| IBIS file generated by  Version 3.24
|   DRA78x_abf
[IBIS ver]   5.0
[File name]   DRA78x_abf.ibs
[File Rev]   1.1.2
[Date]   Tue Aug 30, 2016, 13:57:0
[Source]   Data created at Texas Instruments
[Notes]   DRA78x 15mm IBIS Model Revision History
   Version 1.1.2, August 30th, 2016
   - Combined DDR selectors for similiar signals
   - Modified model names for easier selection
   Version 1.1.1, January 15th, 2015
   - Assign DDR_CK and DDR_NCK as differential pair
   Version 1.1.0, November 7th, 2014
   - Added support for DDR2 and LPDDR2
   Version 1.0.0, May 22, 2014
   - Initial Release
   Note 1) Checked by IBISCHK5.
   Note 2) Interfaces Included in this IBIS Model
   - VIP
   - DPI
   - CAM
   - CPI
   - CSI2
   - EMIF
   - GPMC
   - TIMER
   - I2C
   - UART
   - MCSPI
   - QSPI
   - MCASP
   - DCAN
   - GMAC
   - EMMC
   - GPIO
   - PWM
   - DEBUG
[Disclaimer] Please be aware that in the absence of a written agreement,
   Texas Instruments (TI) assumes no liability for: 1) the
   accuracy of the IBIS models provided to your company, 2) the
   proper functioning of these IBIS models in your design or for
   any resulting applications, or, 3) infringement of patents,
   copyrights, or intellectual property rights resulting from
   your use of these IBIS models. TI provides IBIS models as a
   service to our customers and therefore reserves the right to
   limit distribution of the IBIS models.
[Copyright]   Property of Texas Instruments Incorporated. Unauthorised
   reproduction and/or distribution is strictly prohibited. This
   product is protected under copyright law and trade secret law
   as an unpublished work. Created 2013,(C) Copyright 2013,
   Texas Instruments Incorporated., All Rights Reserved. These
   commodities are under the U.S. Government distribution license
   control.As such,they are not to be re-exported without the
   prior approval of the U.S. Department of Commerce.
|   Component DRA78x_abf
[Component]   DRA78x_abf
[Manufacturer]   Texas Instruments.
| Source IO level model revisions
|Model   Revision   Date
|DDR_DIFFIOPB_V   2.5   23 May 2014
|BC1833DV40DCPBFBP1811_SSCEV   2.0   Sep 11, 2013
|IHHV1833DVHYP1811_SSCEV   1.0   Dec 24, 2012
|BI2C1833DVFZP18_SSCEV   2.0   Sep 11, 2013
|BC1833DV40DCPBFBP1811_SSCEH   2.0   Sep 11, 2013
|CAMERARX_CORE   0.9   March 31, 2014
|DDR_SEIOPB_V   2.5   23 May 2014
|IQ1833DVTCKPBFBP18LL_SSCEV   2.0   Sep 11, 2013
|CAMERARX_ADDON   0.9   March 31, 2014
[Package]
|   typ   min   max
R_pkg   0.667349380701754   64.242E-3   1671.14E-3
L_pkg   3.85005961842105E-009 0.900514E-9   6.82372E-9
C_pkg   5.31210293859649E-013 0.214455E-12   0.846797E-12
[Pin]   signal_name   model_name   R_pin   L_pin   C_pin
P19   ADC_IN6   NC
M22   ADC_IN3   NC
M19   ADC_IN0   NC
P20   ADC_VREFP   NC
M20   ADC_IN1   NC
N22   ADC_IN4   NC
N21   ADC_IN5   NC
M21   ADC_IN2   NC
P18   ADC_IN7   NC
A21   ATESTV   NC
A16   CSI2_0_DX4   Selector_14  866.498E-3 4.24036E-9 0.371535E-12
A15   CSI2_0_DX3   Selector_14  824.084E-3 4.09623E-9 0.353901E-12
B12   CSI2_0_DY1   Selector_7   880.169E-3 3.81411E-9 0.40211E-12
A13   CSI2_0_DX2   Selector_5   917.025E-3 4.11456E-9 0.365851E-12
B15   CSI2_0_DY3   Selector_8   864.002E-3 3.95726E-9 0.383183E-12
B11   CSI2_0_DY0   Selector_8   881.601E-3 3.85263E-9 0.418142E-12
B13   CSI2_0_DY2   Selector_7   810.956E-3 3.78817E-9 0.380345E-12
A12   CSI2_0_DX1   Selector_5   842.043E-3 3.90631E-9 0.371721E-12
A11   CSI2_0_DX0   Selector_14  843.258E-3 3.98139E-9 0.381546E-12
B16   CSI2_0_DY4   Selector_8   880.712E-3 4.08429E-9 0.380274E-12
P17   CVIDEO_VFB   NC
T17   CVIDEO_TVOUT   NC
T18   CVIDEO_RSET   NC
N5   DCAN1_TX   Selector_9   221.153E-3 2.4896E-9  0.508994E-12
N6   DCAN1_RX   Selector_9   174.193E-3 2.2145E-9  0.51767E-12
W6   DCAN2_RX   Selector_4   404.154E-3 4.83175E-9 0.778223E-12
W7   DCAN2_TX   Selector_4   192.368E-3 2.60394E-9 0.469083E-12
W22   DDR1_D30   Selector_3   1303.09E-3 4.54181E-9 0.726069E-12
Y5   DDR1_D5   Selector_3   1117.89E-3 4.60346E-9 0.559528E-12
F1   DDR1_RASN   Selector_11  1296.71E-3 4.52967E-9 0.754591E-12
Y2   DDR1_D22   Selector_3   1482.08E-3 6.2409E-9  0.654749E-12
AB9   DDR1_ECC_D7   Selector_3   1318.63E-3 4.88449E-9 0.563531E-12
W21   DDR1_DQM3   Selector_11  1456.76E-3 4.87842E-9 0.653267E-12
R2   DDR1_A14   Selector_11  1366.99E-3 5.45703E-9 0.784996E-12
U20   DDR1_D27   Selector_3   1251.59E-3 4.23052E-9 0.739335E-12
Y21   DDR1_D9   Selector_3   1410.24E-3 6.0268E-9  0.671587E-12
AA4   DDR1_D6   Selector_3   1162.31E-3 4.7233E-9  0.543846E-12
D2   DDR1_BA2   Selector_11  1345.76E-3 5.19955E-9 0.639721E-12
Y1   DDR1_D23   Selector_3   1408.11E-3 6.15406E-9 0.588347E-12
R22   DDR1_D28   Selector_3   1320.57E-3 4.76807E-9 0.489006E-12
AA9   DDR1_ECC_D6   Selector_3   1365.05E-3 4.86342E-9 0.607781E-12
AA6   DDR1_D0   Selector_3   1059.66E-3 3.64899E-9 0.498846E-12
T22   DDR1_DQSN3   Selector_13  1213.01E-3 5.45946E-9 0.503501E-12
U4   DDR1_A0   Selector_11  1344.44E-3 4.91464E-9 0.702976E-12
N2   DDR1_A7   Selector_11  1428.38E-3 4.75993E-9 0.706672E-12
C3   DDR1_A13   Selector_11  1361.06E-3 5.06314E-9 0.799988E-12
AA21   DDR1_D10   Selector_3   1467.96E-3 6.31542E-9 0.547716E-12
AA8   DDR1_D1   Selector_3   945.134E-3 3.4619E-9  0.630603E-12
AA7   DDR1_D3   Selector_3   957.149E-3 3.58448E-9 0.583994E-12
AB11   DDR1_ECC_D5   Selector_3   1288.72E-3 4.87133E-9 0.699912E-12
AB3   DDR1_DQM2   Selector_11  1231.76E-3 5.08662E-9 0.503327E-12
Y3   DDR1_D18   Selector_3   1232.03E-3 4.85881E-9 0.631657E-12
F3   DDR1_CKE0   Selector_11  1309.3E-3  4.76705E-9 0.661629E-12
AB5   DDR1_DQSN0   Selector_13  1049.22E-3 4.99231E-9 0.470641E-12
D3   DDR1_A2   Selector_11  1451.79E-3 5.79785E-9 0.671604E-12
Y9   DDR1_ECC_D3   Selector_3   1229.56E-3 4.83423E-9 0.735586E-12
AA19   DDR1_D12   Selector_3   1439.57E-3 5.39046E-9 0.68973E-12
V1   DDR1_A15   Selector_11  1671.14E-3 6.82372E-9 0.584748E-12
Y22   DDR1_D11   Selector_3   1477.72E-3 5.88672E-9 0.66686E-12
AA2   DDR1_D17   Selector_3   1345.48E-3 5.16009E-9 0.660701E-12
C1   DDR1_A1   Selector_11  1461.14E-3 6.3818E-9  0.45563E-12
R4   DDR1_A3   Selector_11  1197.34E-3 4.46899E-9 0.55908E-12
AB4   DDR1_D4   Selector_3   1257.55E-3 5.2014E-9  0.502406E-12
AA3   DDR1_D16   Selector_3   1260.55E-3 5.10575E-9 0.591139E-12
AA5   DDR1_DQS0   Selector_15  1095.27E-3 5.06071E-9 0.461046E-12
U3   DDR1_D20   Selector_3   1373.61E-3 5.35193E-9 0.615526E-12
AA13   DDR1_ECC_D4   Selector_3   1323.91E-3 4.88968E-9 0.72932E-12
R3   DDR1_A11   Selector_11  1401.24E-3 5.13832E-9 0.846797E-12
AA10   DDR1_DQS_ECC   Selector_15  1216.87E-3 5.36065E-9 0.556044E-12
D1   DDR1_A10   Selector_11  1329.72E-3 5.13668E-9 0.654383E-12
Y20   DDR1_DQSN1   Selector_13  1342.47E-3 5.82752E-9 0.510552E-12
U22   DDR1_D31   Selector_3   1275.16E-3 4.04716E-9 0.698905E-12
B3   DDR1_BA0   Selector_11  1400.57E-3 6.05502E-9 0.525495E-12
Y11   DDR1_ECC_D0   Selector_3   1389.08E-3 4.76944E-9 0.677831E-12
G2   DDR1_NCK   Selector_12  1342.99E-3 5.99964E-9 0.561576E-12
G1   DDR1_CK   Selector_10  1310.97E-3 5.71231E-9 0.561547E-12
AB20   DDR1_D13   Selector_3   1411.85E-3 5.50356E-9 0.654257E-12
E3   DDR1_WEN   Selector_11  1243.69E-3 4.61238E-9 0.658685E-12
T1   DDR1_A8   Selector_11  1304.21E-3 4.85445E-9 0.734575E-12
V2   DDR1_D19   Selector_3   1371.08E-3 5.42143E-9 0.606473E-12
U2   DDR1_A12   Selector_11  1542.41E-3 5.63849E-9 0.829165E-12
AA12   DDR1_ECC_D1   Selector_3   1144.49E-3 4.56631E-9 0.700588E-12
Y8   DDR1_D2   Selector_3   1013.88E-3 3.94703E-9 0.557904E-12
AA20   DDR1_DQS1   Selector_15  1228.33E-3 5.79816E-9 0.471177E-12
AA11   DDR1_ECC_D2   Selector_3   1220.61E-3 4.58017E-9 0.693337E-12
T21   DDR1_DQS3   Selector_15  1153.95E-3 5.24704E-9 0.550448E-12
Y6   DDR1_D7   Selector_3   1093.76E-3 4.50306E-9 0.494525E-12
V20   DDR1_D29   Selector_3   1164.32E-3 4.20118E-9 0.57292E-12
A3   DDR1_BA1   Selector_11  1458.59E-3 5.71787E-9 0.715307E-12
R21   DDR1_D26   Selector_3   1257.83E-3 5.0006E-9  0.530122E-12
AB18   DDR1_D15   Selector_3   1249.3E-3  4.97423E-9 0.581239E-12
T2   DDR1_A6   Selector_11  1416.66E-3 5.20489E-9 0.708511E-12
Y18   DDR1_DQM1   Selector_11  1284.23E-3 4.79732E-9 0.50954E-12
V3   DDR1_D21   Selector_3   1264.57E-3 4.95585E-9 0.550028E-12
Y17   DDR1_D14   Selector_3   1330.64E-3 5.30397E-9 0.518058E-12
AB10   DDR1_DQSN_ECC   Selector_13  1157.81E-3 5.29728E-9 0.552246E-12
W1   DDR1_DQS2   Selector_15  1243.23E-3 6.03074E-9 0.523353E-12
F2   DDR1_CASN   Selector_11  1359.06E-3 4.84573E-9 0.69557E-12
N3   DDR1_A5   Selector_11  1256.87E-3 4.88274E-9 0.822611E-12
T4   DDR1_A4   Selector_11  1225.96E-3 4.48501E-9 0.686864E-12
N1   DDR1_RST   Selector_11  1200.46E-3 4.86402E-9 0.785997E-12
T20   DDR1_D25   Selector_3   1192.14E-3 4.07414E-9 0.613975E-12
P2   DDR1_ODT0   Selector_11  1319.42E-3 4.7618E-9  0.67937E-12
B2   DDR1_CSN0   Selector_11  1118.13E-3 4.60514E-9 0.624304E-12
U1   DDR1_A9   Selector_11  1430.76E-3 5.46625E-9 0.726337E-12
AB8   DDR1_DQM0   Selector_11  1220.87E-3 4.17469E-9 0.549437E-12
W2   DDR1_DQSN2   Selector_13  1247.14E-3 6.0081E-9  0.5286E-12
U21   DDR1_D24   Selector_3   1331.68E-3 4.36055E-9 0.733678E-12
AB13   DDR1_DQM_ECC   Selector_11  1291.15E-3 4.6118E-9  0.626638E-12
AA18   DDR1_D8   Selector_3   1418.02E-3 5.43567E-9 0.642913E-12
H1   EMU0   Selector_9   346.558E-3 3.945E-9   0.481326E-12
H2   EMU1   Selector_9   273.662E-3 3.26523E-9 0.455933E-12
C8   GPMC_CS6   Selector_4   284.574E-3 3.07589E-9 0.456596E-12
B4   GPMC_AD14   Selector_4   370.025E-3 4.53157E-9 0.506776E-12
F8   GPMC_AD2   Selector_4   247.733E-3 2.79628E-9 0.40664E-12
A5   GPMC_AD9   Selector_4   420.627E-3 4.64798E-9 0.533623E-12
D10   GPMC_CS2   Selector_4   187.985E-3 2.10165E-9 0.402136E-12
A4   GPMC_AD15   Selector_4   397.46E-3  4.86112E-9 0.54337E-12
A10   GPMC_OEN_REN   Selector_4   373.838E-3 3.74242E-9 0.451922E-12
C12   GPMC_CLK   Selector_4   326.387E-3 3.50172E-9 0.618617E-12
E8   GPMC_AD0   Selector_4   267.003E-3 2.80033E-9 0.441078E-12
D8   GPMC_WAIT0   Selector_4   266.22E-3  2.88134E-9 0.40446E-12
D6   GPMC_AD10   Selector_4   221.234E-3 2.54407E-9 0.422159E-12
C10   GPMC_CS0   Selector_4   311.079E-3 3.00524E-9 0.44399E-12
E12   GPMC_BEN1   Selector_4   320.958E-3 3.02188E-9 0.594246E-12
A6   GPMC_AD4   Selector_4   437.778E-3 4.50088E-9 0.532669E-12
D12   GPMC_BEN0   Selector_4   292.929E-3 3.06566E-9 0.606716E-12
D7   GPMC_AD13   Selector_4   304.94E-3  3.19335E-9 0.404685E-12
C6   GPMC_AD7   Selector_4   318.071E-3 3.30116E-9 0.469481E-12
F7   GPMC_AD5   Selector_4   185.525E-3 2.0225E-9  0.416218E-12
C5   GPMC_AD11   Selector_4   325.471E-3 3.54687E-9 0.491936E-12
F10   GPMC_CS5   Selector_4   64.242E-3  0.900514E-9 0.269895E-12
F12   GPMC_ADVN_ALE   Selector_4   266.228E-3 3.02405E-9 0.433779E-12
B9   GPMC_CS4   Selector_4   335.103E-3 3.42038E-9 0.495123E-12
B10   GPMC_WEN   Selector_4   347.42E-3  3.76872E-9 0.466852E-12
B6   GPMC_AD8   Selector_4   330.979E-3 3.67024E-9 0.516724E-12
A7   GPMC_AD1   Selector_4   356.051E-3 4.20904E-9 0.431934E-12
B5   GPMC_AD12   Selector_4   348.127E-3 3.95513E-9 0.545603E-12
E7   GPMC_AD6   Selector_4   170.88E-3  1.99455E-9 0.378953E-12
B7   GPMC_AD3   Selector_4   324.465E-3 3.66337E-9 0.443124E-12
A9   GPMC_CS3   Selector_4   361.691E-3 3.93006E-9 0.505481E-12
E10   GPMC_CS1   Selector_4   175.122E-3 1.66792E-9 0.3576E-12
L3   I2C1_SCL   Selector_6   253.012E-3 2.73735E-9 0.427091E-12
L6   I2C2_SCL   Selector_6   75.9648E-3 0.951563E-9 0.319419E-12
L5   I2C2_SDA   Selector_6   125.18E-3  1.32917E-9 0.429362E-12
L4   I2C1_SDA   Selector_6   200.127E-3 2.27796E-9 0.471893E-12
B17   MDIO_D   Selector_4   344.949E-3 4.04087E-9 0.518979E-12
B19   MDIO_MCLK   Selector_4   350.85E-3  4.29974E-9 0.567622E-12
G5   NMIN   Selector_2   206.034E-3 2.38103E-9 0.441195E-12
G3   PORZ   Selector_16  262.543E-3 3.23109E-9 0.436378E-12
G4   RESETN   Selector_2   221.901E-3 2.67053E-9 0.416783E-12
F17   RGMII0_TXD0   Selector_4   190.61E-3  2.90538E-9 0.453282E-12
E17   RGMII0_TXD1   Selector_4   243.515E-3 2.63118E-9 0.416182E-12
C16   RGMII0_TXC   Selector_4   241.728E-3 2.9564E-9  0.393586E-12
A20   RGMII0_RXD0   Selector_4   378.744E-3 5.06456E-9 0.540103E-12
D16   RGMII0_TXD2   Selector_4   272.921E-3 3.27597E-9 0.364109E-12
C18   RGMII0_RXCTL   Selector_4   334.922E-3 3.70159E-9 0.476584E-12
B18   RGMII0_RXC   Selector_4   383.991E-3 4.38625E-9 0.584646E-12
C17   RGMII0_TXCTL   Selector_4   299.95E-3  3.2778E-9  0.45012E-12
A19   RGMII0_RXD3   Selector_4   382.21E-3  4.86108E-9 0.516381E-12
C20   RGMII0_RXD1   Selector_4   337.059E-3 4.59601E-9 0.437991E-12
B20   RGMII0_RXD2   Selector_4   337.895E-3 4.50338E-9 0.543729E-12
E16   RGMII0_TXD3   Selector_4   258.565E-3 2.83197E-9 0.371553E-12
F4   RSTOUTN   Selector_17  380.521E-3 4.67151E-9 0.614741E-12
J6   RTCK   Selector_17  116.119E-3 1.272E-9   0.297361E-12
T5   SPI1_D0   Selector_9   400.982E-3 4.51214E-9 0.798667E-12
M2   SPI1_SCLK   Selector_9   267.537E-3 2.74861E-9 0.533728E-12
U6   SPI1_D1   Selector_9   264.657E-3 3.64443E-9 0.560725E-12
R5   SPI1_CS1   Selector_9   343.795E-3 3.60294E-9 0.730371E-12
R6   SPI1_CS0   Selector_9   184.528E-3 2.64387E-9 0.507092E-12
L2   SPI2_CS0   Selector_9   258.507E-3 3.05366E-9 0.398683E-12
N4   SPI2_D1   Selector_9   159.815E-3 1.82356E-9 0.50115E-12
L1   SPI2_SCLK   Selector_9   350.336E-3 3.8191E-9  0.466382E-12
R7   SPI2_D0   Selector_9   194.814E-3 2.55749E-9 0.476249E-12
J2   TCLK   Selector_1   254.697E-3 3.15214E-9 0.378464E-12
J1   TDI   Selector_2   326.413E-3 3.56361E-9 0.460549E-12
J4   TDO   Selector_17  149.34E-3  1.81311E-9 0.321612E-12
J3   TMS   Selector_2   263.583E-3 2.96504E-9 0.445849E-12
J5   TRSTN   Selector_2   140.82E-3  1.56546E-9 0.304121E-12
C14   UART1_RTSN   Selector_4   271.077E-3 3.37526E-9 0.592546E-12
E14   UART1_TXD   Selector_4   264.17E-3  3.29024E-9 0.580159E-12
F14   UART1_CTSN   Selector_4   186.167E-3 2.17244E-9 0.522293E-12
F13   UART1_RXD   Selector_4   183.573E-3 2.09803E-9 0.458722E-12
F16   UART2_RTSN   Selector_4   324.1E-3   3.89433E-9 0.569445E-12
D14   UART2_RXD   Selector_4   355.638E-3 3.93152E-9 0.716287E-12
F15   UART2_CTSN   Selector_4   294.057E-3 3.59825E-9 0.5892E-12
D15   UART2_TXD   Selector_4   282.377E-3 3.48879E-9 0.582841E-12
G18   VIN1A_D0   Selector_9   243.254E-3 2.85171E-9 0.501809E-12
K21   VIN1A_D10   Selector_9   305.782E-3 3.65235E-9 0.458586E-12
G19   VIN1A_VSYNC0   Selector_9   246.63E-3  3.12189E-9 0.492055E-12
J17   VIN1A_D8   Selector_9   228.648E-3 2.7531E-9  0.442602E-12
K17   VIN1A_D12   Selector_9   176.785E-3 2.20565E-9 0.388461E-12
G21   VIN1A_D1   Selector_9   363.135E-3 4.19976E-9 0.575956E-12
F22   VIN1A_CLK0   Selector_9   392.642E-3 4.6109E-9  0.584552E-12
K22   VIN1A_D9   Selector_9   322.551E-3 4.1764E-9  0.421938E-12
H22   VIN1A_D6   Selector_9   377.875E-3 4.39918E-9 0.51729E-12
G22   VIN1A_D2   Selector_9   377.7E-3   4.53068E-9 0.560377E-12
K18   VIN1A_D11   Selector_9   140.113E-3 1.67467E-9 0.346405E-12
F19   VIN1A_HSYNC0   Selector_9   284.459E-3 3.30938E-9 0.524099E-12
K19   VIN1A_D13   Selector_9   199.308E-3 2.30236E-9 0.395571E-12
K20   VIN1A_D14   Selector_9   225.717E-3 2.61957E-9 0.370053E-12
H19   VIN1A_D5   Selector_9   237.915E-3 2.77378E-9 0.458354E-12
F20   VIN1A_FLD0   Selector_9   301.259E-3 3.71239E-9 0.51085E-12
L21   VIN1A_D15   Selector_9   299.827E-3 3.51197E-9 0.45532E-12
F21   VIN1A_DE0   Selector_9   358.032E-3 4.33398E-9 0.519573E-12
H20   VIN1A_D4   Selector_9   261.044E-3 3.17335E-9 0.468927E-12
H21   VIN1A_D7   Selector_9   336.581E-3 3.95216E-9 0.508497E-12
H18   VIN1A_D3   Selector_9   318.602E-3 3.64388E-9 0.577444E-12
M18   VIN2A_FLD0   Selector_9   107.879E-3 1.39908E-9 0.25939E-12
M17   VIN2A_DE0   Selector_9   69.4518E-3 0.993642E-9 0.214455E-12
L22   VIN2A_CLK0   Selector_9   326.657E-3 4.13124E-9 0.457766E-12
U15   VOUT1_D2   Selector_4   188.192E-3 2.06593E-9 0.524972E-12
U17   VOUT1_DE   Selector_4   180.267E-3 2.5353E-9  0.421769E-12
W8   VOUT1_D21   Selector_4   286.194E-3 3.22952E-9 0.660641E-12
W9   VOUT1_D19   Selector_4   176.719E-3 2.32055E-9 0.469196E-12
W11   VOUT1_D17   Selector_4   170.859E-3 1.88713E-9 0.475399E-12
U13   VOUT1_D10   Selector_4   121.41E-3  1.22509E-9 0.414317E-12
V9   VOUT1_D18   Selector_4   188.281E-3 2.08068E-9 0.521271E-12
AB17   VOUT1_CLK   Selector_4   365.568E-3 4.16017E-9 0.565211E-12
U9   VOUT1_D16   Selector_4   183.337E-3 2.11554E-9 0.534405E-12
AA15   VOUT1_D6   Selector_4   388.553E-3 3.79821E-9 0.620296E-12
AA17   VOUT1_HSYNC   Selector_4   406.915E-3 4.58133E-9 0.582066E-12
W16   VOUT1_D0   Selector_4   249.496E-3 2.74357E-9 0.544844E-12
AB15   VOUT1_D7   Selector_4   407.232E-3 4.46019E-9 0.539498E-12
AA14   VOUT1_D8   Selector_4   343.58E-3  3.34818E-9 0.554761E-12
W13   VOUT1_D13   Selector_4   238.288E-3 2.20297E-9 0.483663E-12
W15   VOUT1_D5   Selector_4   270.299E-3 2.89534E-9 0.543448E-12
W17   VOUT1_FLD   Selector_4   392.595E-3 4.29688E-9 0.619062E-12
AB14   VOUT1_D9   Selector_4   375.782E-3 3.99293E-9 0.57511E-12
U11   VOUT1_D14   Selector_4   91.4322E-3 0.938044E-9 0.395492E-12
Y15   VOUT1_D4   Selector_4   275.703E-3 3.09509E-9 0.440349E-12
V16   VOUT1_D1   Selector_4   249.155E-3 2.69511E-9 0.49623E-12
Y13   VOUT1_D12   Selector_4   243.754E-3 2.47516E-9 0.457168E-12
V11   VOUT1_D15   Selector_4   146.232E-3 1.44691E-9 0.461628E-12
U16   VOUT1_VSYNC   Selector_4   221.18E-3  2.43907E-9 0.495724E-12
V7   VOUT1_D23   Selector_4   193.825E-3 2.65994E-9 0.580721E-12
U7   VOUT1_D22   Selector_4   185.923E-3 2.5291E-9  0.426436E-12
V13   VOUT1_D11   Selector_4   106.384E-3 1.20262E-9 0.365368E-12
V15   VOUT1_D3   Selector_4   172.909E-3 2.04259E-9 0.422534E-12
U8   VOUT1_D20   Selector_4   165.759E-3 2.12333E-9 0.545066E-12
B21   XI_OSC1   NC
E22   XI_OSC0   NC
C21   XO_OSC1   NC
D22   XO_OSC0   NC
M1   XREF_CLK0   Selector_9   330.711E-3 3.47713E-9 0.50945E-12
[Diff Pin] inv_pin vdiff tdelay_typ tdelay_min tdelay_max
|Differential signal data for cell CAMERARX_ADDON
|CSI2_0_DX3   CSI2_0_DY3
A15   B15   200m   NA
|CSI2_0_DX4   CSI2_0_DY4
A16   B16   200m   NA
|CSI2_0_DX0   CSI2_0_DY0
A11   B11   200m   NA
|Differential signal data for cell CAMERARX_CORE
|CSI2_0_DX1   CSI2_0_DY1
A12   B12   200m   NA
|CSI2_0_DX2   CSI2_0_DY2
A13   B13   200m   NA
|Differential signal data for cell DDR_DIFFIOPB_V
|DDR1_DQS1   DDR1_DQSN1
AA20   Y20   200m   0
|DDR1_DQS_ECC   DDR1_DQSN_ECC
AA10   AB10   200m   0
|DDR1_CK   DDR1_NCK
G1   G2   200m   0
|DDR1_DQS3   DDR1_DQSN3
T21   T22   200m   0
|DDR1_DQS0   DDR1_DQSN0
AA5   AB5   200m   0
|DDR1_DQS2   DDR1_DQSN2
W1   W2   200m   0
|   Usage INPUT#1.8/3.3###IQ1833DVTCKPBFBP18LL_SSCEV.PAD
|   Base model IQ1833DVTCKPBFBP18LL_SSCEV
[Model Selector] Selector_1
IQ1833_V_10P_1P8_M#1 INPUT,1.8V,1.8V MODE,IND,10 PERCENT%,IQ1833_V_10P_1P8
IQ1833_V_5P_1P8_M#2 INPUT,1.8V,1.8V MODE,IND,5 PERCENT%,IQ1833_V_5P_1P8
IQ1833_V_10P_3P3_M#3 INPUT,3.3V,3.3V MODE,IND,10 PERCENT%,IQ1833_V_10P_3P3
IQ1833_V_5P_3P3_M#4 INPUT,3.3V,3.3V MODE,IND,5 PERCENT%,IQ1833_V_5P_3P3
|   Usage INPUT#1.8/3.3###BC1833DV40DCPBFBP1811_SSCEV.PAD
|   Base model BC1833DV40DCPBFBP1811_SSCEV
[Model Selector] Selector_2
BC40D_V_10P_!SC1_1P8_M#194 I/O,1.8V,40D CLASS MODE FAST MODE,IND,10 PERCENT%,BC40D_V_10P_!SC1_1P8
BC40D_V_10P_SC1_1P8_M#195 I/O,1.8V,40C CLASS MODE SLOW MODE,IND,10 PERCENT%,BC40D_V_10P_SC1_1P8
BC40D_V_5P_!SC1_1P8_M#196 I/O,1.8V,40D CLASS MODE FAST MODE,IND,5 PERCENT%,BC40D_V_5P_!SC1_1P8
BC40D_V_5P_SC1_1P8_M#197 I/O,1.8V,40C CLASS MODE SLOW MODE,IND,5 PERCENT%,BC40D_V_5P_SC1_1P8
BC40D_V_10P_!SC1_3P3_M#198 I/O,3.3V,40D CLASS MODE FAST MODE,IND,10 PERCENT%,BC40D_V_10P_!SC1_3P3
BC40D_V_10P_SC1_3P3_M#199 I/O,3.3V,40C CLASS MODE SLOW MODE,IND,10 PERCENT%,BC40D_V_10P_SC1_3P3
BC40D_V_5P_!SC1_3P3_M#200 I/O,3.3V,40D CLASS MODE FAST MODE,IND,5 PERCENT%,BC40D_V_5P_!SC1_3P3
BC40D_V_5P_SC1_3P3_M#201 I/O,3.3V,40C CLASS MODE SLOW MODE,IND,5 PERCENT%,BC40D_V_5P_SC1_3P3
|   Usage I/O#1.2/1.35/1.5/1.8###DDR_SEIOPB_V.PAD
|   Base model DDR_SEIOPB_V
[Model Selector] Selector_3
SR000_DRV48_1P8_M#100 I/O,1.8V,SR000_DRV48_1P8
SR011_DRV40_1P8_M#101 I/O,1.8V,SR011_DRV40_1P8
SR010_DRV40_1P8_M#102 I/O,1.8V,SR010_DRV40_1P8
SR101_DRV40_1P8_M#103 I/O,1.8V,SR101_DRV40_1P8
SR100_DRV40_1P8_M#104 I/O,1.8V,SR100_DRV40_1P8
SR110_DRV40_1P8_M#105 I/O,1.8V,SR110_DRV40_1P8
SR111_DRV40_1P8_M#106 I/O,1.8V,SR111_DRV40_1P8
SR001_DRV40_1P8_M#107 I/O,1.8V,SR001_DRV40_1P8
SR000_DRV40_1P8_M#108 I/O,1.8V,SR000_DRV40_1P8
SR011_DRV34_1P8_M#109 I/O,1.8V,SR011_DRV34_1P8
SR010_DRV34_1P8_M#110 I/O,1.8V,SR010_DRV34_1P8
SR101_DRV34_1P8_M#111 I/O,1.8V,SR101_DRV34_1P8
SR100_DRV34_1P8_M#112 I/O,1.8V,SR100_DRV34_1P8
SR110_DRV34_1P8_M#113 I/O,1.8V,SR110_DRV34_1P8
SR111_DRV34_1P8_M#114 I/O,1.8V,SR111_DRV34_1P8
SR001_DRV34_1P8_M#115 I/O,1.8V,SR001_DRV34_1P8
SR000_DRV34_1P8_M#116 I/O,1.8V,SR000_DRV34_1P8
DDR3_ODT_80_1P5_M#117 INPUT,1.5V,DDR3_ODT_80_1P5
DDR3_ODT_60_1P5_M#118 INPUT,1.5V,DDR3_ODT_60_1P5
DDR3_ODT_120_1P5_M#119 INPUT,1.5V,DDR3_ODT_120_1P5
DDR3L_ODT_80_1P35_M#120 INPUT,1.35V,DDR3L_ODT_80_1P35
DDR3L_ODT_60_1P35_M#121 INPUT,1.35V,DDR3L_ODT_60_1P35
DDR3L_ODT_120_1P35_M#122 INPUT,1.35V,DDR3L_ODT_120_1P35
DDR2_ODT_120_1P8_M#123 INPUT,1.8V,DDR2_ODT_120_1P8
DDR2_ODT_80_1P8_M#124 INPUT,1.8V,DDR2_ODT_80_1P8
DDR2_ODT_60_1P8_M#125 INPUT,1.8V,DDR2_ODT_60_1P8
SR011_DRV40_1P5_M#126 I/O,1.5V,SR011_DRV40_1P5
SR010_DRV40_1P5_M#127 I/O,1.5V,SR010_DRV40_1P5
SR101_DRV40_1P5_M#128 I/O,1.5V,SR101_DRV40_1P5
SR100_DRV40_1P5_M#129 I/O,1.5V,SR100_DRV40_1P5
SR011_DRV60_1P2_M#13 I/O,1.2V,SR011_DRV60_1P2
SR110_DRV40_1P5_M#130 I/O,1.5V,SR110_DRV40_1P5
SR111_DRV40_1P5_M#131 I/O,1.5V,SR111_DRV40_1P5
SR001_DRV40_1P5_M#132 I/O,1.5V,SR001_DRV40_1P5
SR000_DRV40_1P5_M#133 I/O,1.5V,SR000_DRV40_1P5
SR011_DRV34_1P5_M#134 I/O,1.5V,SR011_DRV34_1P5
SR010_DRV34_1P5_M#135 I/O,1.5V,SR010_DRV34_1P5
SR101_DRV34_1P5_M#136 I/O,1.5V,SR101_DRV34_1P5
SR100_DRV34_1P5_M#137 I/O,1.5V,SR100_DRV34_1P5
SR110_DRV34_1P5_M#138 I/O,1.5V,SR110_DRV34_1P5
SR111_DRV34_1P5_M#139 I/O,1.5V,SR111_DRV34_1P5
SR010_DRV60_1P2_M#14 I/O,1.2V,SR010_DRV60_1P2
SR001_DRV34_1P5_M#140 I/O,1.5V,SR001_DRV34_1P5
SR000_DRV34_1P5_M#141 I/O,1.5V,SR000_DRV34_1P5
SR011_DRV48_1P5_M#142 I/O,1.5V,SR011_DRV48_1P5
SR010_DRV48_1P5_M#143 I/O,1.5V,SR010_DRV48_1P5
SR101_DRV48_1P5_M#144 I/O,1.5V,SR101_DRV48_1P5
SR100_DRV48_1P5_M#145 I/O,1.5V,SR100_DRV48_1P5
SR110_DRV48_1P5_M#146 I/O,1.5V,SR110_DRV48_1P5
SR111_DRV48_1P5_M#147 I/O,1.5V,SR111_DRV48_1P5
SR001_DRV48_1P5_M#148 I/O,1.5V,SR001_DRV48_1P5
SR000_DRV48_1P5_M#149 I/O,1.5V,SR000_DRV48_1P5
SR101_DRV60_1P2_M#15 I/O,1.2V,SR101_DRV60_1P2
SR011_DRV40_1P35_M#150 I/O,1.35V,SR011_DRV40_1P35
SR010_DRV40_1P35_M#151 I/O,1.35V,SR010_DRV40_1P35
SR101_DRV40_1P35_M#152 I/O,1.35V,SR101_DRV40_1P35
SR100_DRV40_1P35_M#153 I/O,1.35V,SR100_DRV40_1P35
SR110_DRV40_1P35_M#154 I/O,1.35V,SR110_DRV40_1P35
SR111_DRV40_1P35_M#155 I/O,1.35V,SR111_DRV40_1P35
SR001_DRV40_1P35_M#156 I/O,1.35V,SR001_DRV40_1P35
SR000_DRV40_1P35_M#157 I/O,1.35V,SR000_DRV40_1P35
SR011_DRV34_1P35_M#158 I/O,1.35V,SR011_DRV34_1P35
SR010_DRV34_1P35_M#159 I/O,1.35V,SR010_DRV34_1P35
SR100_DRV60_1P2_M#16 I/O,1.2V,SR100_DRV60_1P2
SR101_DRV34_1P35_M#160 I/O,1.35V,SR101_DRV34_1P35
SR100_DRV34_1P35_M#161 I/O,1.35V,SR100_DRV34_1P35
SR110_DRV34_1P35_M#162 I/O,1.35V,SR110_DRV34_1P35
SR111_DRV34_1P35_M#163 I/O,1.35V,SR111_DRV34_1P35
SR001_DRV34_1P35_M#164 I/O,1.35V,SR001_DRV34_1P35
SR000_DRV34_1P35_M#165 I/O,1.35V,SR000_DRV34_1P35
SR011_DRV48_1P35_M#166 I/O,1.35V,SR011_DRV48_1P35
SR010_DRV48_1P35_M#167 I/O,1.35V,SR010_DRV48_1P35
SR101_DRV48_1P35_M#168 I/O,1.35V,SR101_DRV48_1P35
SR100_DRV48_1P35_M#169 I/O,1.35V,SR100_DRV48_1P35
SR110_DRV60_1P2_M#17 I/O,1.2V,SR110_DRV60_1P2
SR110_DRV48_1P35_M#170 I/O,1.35V,SR110_DRV48_1P35
SR111_DRV48_1P35_M#171 I/O,1.35V,SR111_DRV48_1P35
SR001_DRV48_1P35_M#172 I/O,1.35V,SR001_DRV48_1P35
SR000_DRV48_1P35_M#173 I/O,1.35V,SR000_DRV48_1P35
SR111_DRV60_1P2_M#18 I/O,1.2V,SR111_DRV60_1P2
SR001_DRV60_1P2_M#19 I/O,1.2V,SR001_DRV60_1P2
SR000_DRV60_1P2_M#20 I/O,1.2V,SR000_DRV60_1P2
SR011_DRV80_1P2_M#29 I/O,1.2V,SR011_DRV80_1P2
SR010_DRV80_1P2_M#30 I/O,1.2V,SR010_DRV80_1P2
SR101_DRV80_1P2_M#31 I/O,1.2V,SR101_DRV80_1P2
SR100_DRV80_1P2_M#32 I/O,1.2V,SR100_DRV80_1P2
SR110_DRV80_1P2_M#33 I/O,1.2V,SR110_DRV80_1P2
SR111_DRV80_1P2_M#34 I/O,1.2V,SR111_DRV80_1P2
SR001_DRV80_1P2_M#35 I/O,1.2V,SR001_DRV80_1P2
SR000_DRV80_1P2_M#36 I/O,1.2V,SR000_DRV80_1P2
SR011_DRV40_1P2_M#45 I/O,1.2V,SR011_DRV40_1P2
SR010_DRV40_1P2_M#46 I/O,1.2V,SR010_DRV40_1P2
SR101_DRV40_1P2_M#47 I/O,1.2V,SR101_DRV40_1P2
SR100_DRV40_1P2_M#48 I/O,1.2V,SR100_DRV40_1P2
SR110_DRV40_1P2_M#49 I/O,1.2V,SR110_DRV40_1P2
SR111_DRV40_1P2_M#50 I/O,1.2V,SR111_DRV40_1P2
SR001_DRV40_1P2_M#51 I/O,1.2V,SR001_DRV40_1P2
SR000_DRV40_1P2_M#52 I/O,1.2V,SR000_DRV40_1P2
SR011_DRV34_1P2_M#53 I/O,1.2V,SR011_DRV34_1P2
SR010_DRV34_1P2_M#54 I/O,1.2V,SR010_DRV34_1P2
SR101_DRV34_1P2_M#55 I/O,1.2V,SR101_DRV34_1P2
SR100_DRV34_1P2_M#56 I/O,1.2V,SR100_DRV34_1P2
SR110_DRV34_1P2_M#57 I/O,1.2V,SR110_DRV34_1P2
SR111_DRV34_1P2_M#58 I/O,1.2V,SR111_DRV34_1P2
SR001_DRV34_1P2_M#59 I/O,1.2V,SR001_DRV34_1P2
SR000_DRV34_1P2_M#60 I/O,1.2V,SR000_DRV34_1P2
SR011_DRV48_1P2_M#77 I/O,1.2V,SR011_DRV48_1P2
SR010_DRV48_1P2_M#78 I/O,1.2V,SR010_DRV48_1P2
SR101_DRV48_1P2_M#79 I/O,1.2V,SR101_DRV48_1P2
SR100_DRV48_1P2_M#80 I/O,1.2V,SR100_DRV48_1P2
SR110_DRV48_1P2_M#81 I/O,1.2V,SR110_DRV48_1P2
SR111_DRV48_1P2_M#82 I/O,1.2V,SR111_DRV48_1P2
SR001_DRV48_1P2_M#83 I/O,1.2V,SR001_DRV48_1P2
SR000_DRV48_1P2_M#84 I/O,1.2V,SR000_DRV48_1P2
SR011_DRV48_1P8_M#93 I/O,1.8V,SR011_DRV48_1P8
SR010_DRV48_1P8_M#94 I/O,1.8V,SR010_DRV48_1P8
SR101_DRV48_1P8_M#95 I/O,1.8V,SR101_DRV48_1P8
SR100_DRV48_1P8_M#96 I/O,1.8V,SR100_DRV48_1P8
SR110_DRV48_1P8_M#97 I/O,1.8V,SR110_DRV48_1P8
SR111_DRV48_1P8_M#98 I/O,1.8V,SR111_DRV48_1P8
SR001_DRV48_1P8_M#99 I/O,1.8V,SR001_DRV48_1P8
|   Usage I/O#1.8/3.3###BC1833DV40DCPBFBP1811_SSCEH.PAD
|   Base model BC1833DV40DCPBFBP1811_SSCEH
[Model Selector] Selector_4
BC40D_H_10P_!SC1_1P8_M#182 I/O,1.8V,40D CLASS MODE FAST MODE,IND,10 PERCENT%,BC40D_H_10P_!SC1_1P8
BC40D_H_10P_SC1_1P8_M#183 I/O,1.8V,40C CLASS MODE SLOW MODE,IND,10 PERCENT%,BC40D_H_10P_SC1_1P8
BC40D_H_5P_!SC1_1P8_M#184 I/O,1.8V,40D CLASS MODE FAST MODE,IND,5 PERCENT%,BC40D_H_5P_!SC1_1P8
BC40D_H_5P_SC1_1P8_M#185 I/O,1.8V,40C CLASS MODE SLOW MODE,IND,5 PERCENT%,BC40D_H_5P_SC1_1P8
BC40D_H_10P_!SC1_3P3_M#186 I/O,3.3V,40D CLASS MODE FAST MODE,IND,10 PERCENT%,BC40D_H_10P_!SC1_3P3
BC40D_H_10P_SC1_3P3_M#187 I/O,3.3V,40C CLASS MODE SLOW MODE,IND,10 PERCENT%,BC40D_H_10P_SC1_3P3
BC40D_H_5P_!SC1_3P3_M#188 I/O,3.3V,40D CLASS MODE FAST MODE,IND,5 PERCENT%,BC40D_H_5P_!SC1_3P3
BC40D_H_5P_SC1_3P3_M#189 I/O,3.3V,40C CLASS MODE SLOW MODE,IND,5 PERCENT%,BC40D_H_5P_SC1_3P3
|   Usage INPUT#1.8###CAMERARX_CORE.PADP
|   Base model CAMERARX_CORE
[Model Selector] Selector_5
CAMERARX_CORE_HSRX_M#176 INPUT,1.8V,CAMERARX_CORE_HSRX
CAMERARX_CORE_LPRX_M#177 INPUT,1.8V,CAMERARX_CORE_LPRX
CAMERARX_CORE_ULPRX_M#178 INPUT,1.8V,CAMERARX_CORE_ULPRX
CAMERARX_CORE_PD_ON_M#179 INPUT,1.8V,CAMERARX_CORE_PD_ON
CAMERARX_CORE_PU_ON_M#180 INPUT,1.8V,CAMERARX_CORE_PU_ON
CAMERARX_CORE_PUPD0_M#181 INPUT,1.8V,CAMERARX_CORE_PUPD0
|   Usage I/O#1.8/3.3###BI2C1833DVFZP18_SSCEV.PAD
|   Base model BI2C1833DVFZP18_SSCEV
[Model Selector] Selector_6
FAST_STD_MODE_1.8V_10P_1P8_M#190 I/O_OPEN_DRAIN,1.8V,FAST MODE AND STD MODE,IND,10 PERCENT%,FAST_STD_MODE_1.8V_10P_1P8
FAST_STD_MODE_3.3V_10P_3P3_M#191 I/O_OPEN_DRAIN,3.3V,FAST MODE AND STD MODE,IND,10 PERCENT%,FAST_STD_MODE_3.3V_10P_3P3
FAST_STD_MODE_1.8V_5P_1P8_M#192 I/O_OPEN_DRAIN,1.8V,FAST MODE AND STD MODE,IND,5 PERCENT%,FAST_STD_MODE_1.8V_5P_1P8
FAST_STD_MODE_3.3V_5P_3P3_M#193 I/O_OPEN_DRAIN,3.3V,FAST MODE AND STD MODE,IND,5 PERCENT%,FAST_STD_MODE_3.3V_5P_3P3
|   Usage INPUT#1.8###CAMERARX_CORE.PADN
|   Base model CAMERARX_CORE
[Model Selector] Selector_7
CAMERARX_CORE_HSRX_M#176 INPUT,1.8V,CAMERARX_CORE_HSRX
CAMERARX_CORE_LPRX_M#177 INPUT,1.8V,CAMERARX_CORE_LPRX
CAMERARX_CORE_ULPRX_M#178 INPUT,1.8V,CAMERARX_CORE_ULPRX
CAMERARX_CORE_PD_ON_M#179 INPUT,1.8V,CAMERARX_CORE_PD_ON
CAMERARX_CORE_PU_ON_M#180 INPUT,1.8V,CAMERARX_CORE_PU_ON
CAMERARX_CORE_PUPD0_M#181 INPUT,1.8V,CAMERARX_CORE_PUPD0
|   Usage INPUT#1.8###CAMERARX_ADDON.PADN
|   Base model CAMERARX_ADDON
[Model Selector] Selector_8
CAMERARX_ADDON_PD_ON_M#10 INPUT,1.8V,CAMERARX_ADDON_PD_ON
CAMERARX_ADDON_PU_ON_M#11 INPUT,1.8V,CAMERARX_ADDON_PU_ON
CAMERARX_ADDON_PUPD0_M#12 INPUT,1.8V,CAMERARX_ADDON_PUPD0
CAMERARX_ADDON_HSRX_M#7 INPUT,1.8V,CAMERARX_ADDON_HSRX
CAMERARX_ADDON_LPRX_M#8 INPUT,1.8V,CAMERARX_ADDON_LPRX
CAMERARX_ADDON_ULPRX_M#9 INPUT,1.8V,CAMERARX_ADDON_ULPRX
|   Usage I/O#1.8/3.3###BC1833DV40DCPBFBP1811_SSCEV.PAD
|   Base model BC1833DV40DCPBFBP1811_SSCEV
[Model Selector] Selector_9
BC40D_V_10P_!SC1_1P8_M#194 I/O,1.8V,40D CLASS MODE FAST MODE,IND,10 PERCENT%,BC40D_V_10P_!SC1_1P8
BC40D_V_10P_SC1_1P8_M#195 I/O,1.8V,40C CLASS MODE SLOW MODE,IND,10 PERCENT%,BC40D_V_10P_SC1_1P8
BC40D_V_5P_!SC1_1P8_M#196 I/O,1.8V,40D CLASS MODE FAST MODE,IND,5 PERCENT%,BC40D_V_5P_!SC1_1P8
BC40D_V_5P_SC1_1P8_M#197 I/O,1.8V,40C CLASS MODE SLOW MODE,IND,5 PERCENT%,BC40D_V_5P_SC1_1P8
BC40D_V_10P_!SC1_3P3_M#198 I/O,3.3V,40D CLASS MODE FAST MODE,IND,10 PERCENT%,BC40D_V_10P_!SC1_3P3
BC40D_V_10P_SC1_3P3_M#199 I/O,3.3V,40C CLASS MODE SLOW MODE,IND,10 PERCENT%,BC40D_V_10P_SC1_3P3
BC40D_V_5P_!SC1_3P3_M#200 I/O,3.3V,40D CLASS MODE FAST MODE,IND,5 PERCENT%,BC40D_V_5P_!SC1_3P3
BC40D_V_5P_SC1_3P3_M#201 I/O,3.3V,40C CLASS MODE SLOW MODE,IND,5 PERCENT%,BC40D_V_5P_SC1_3P3
|   Usage OUTPUT#1.2/1.35/1.5/1.8###DDR_DIFFIOPB_V.PADP
|   Base model DDR_DIFFIOPB_V
[Model Selector] Selector_10
SR011_DRV60_1P2_M#202 I/O,1.2V,SR011_DRV60_1P2
SR010_DRV60_1P2_M#203 I/O,1.2V,SR010_DRV60_1P2
SR101_DRV60_1P2_M#204 I/O,1.2V,SR101_DRV60_1P2
SR100_DRV60_1P2_M#205 I/O,1.2V,SR100_DRV60_1P2
SR110_DRV60_1P2_M#206 I/O,1.2V,SR110_DRV60_1P2
SR111_DRV60_1P2_M#207 I/O,1.2V,SR111_DRV60_1P2
SR001_DRV60_1P2_M#208 I/O,1.2V,SR001_DRV60_1P2
SR000_DRV60_1P2_M#209 I/O,1.2V,SR000_DRV60_1P2
SR011_DRV80_1P2_M#218 I/O,1.2V,SR011_DRV80_1P2
SR010_DRV80_1P2_M#219 I/O,1.2V,SR010_DRV80_1P2
SR101_DRV80_1P2_M#220 I/O,1.2V,SR101_DRV80_1P2
SR100_DRV80_1P2_M#221 I/O,1.2V,SR100_DRV80_1P2
SR110_DRV80_1P2_M#222 I/O,1.2V,SR110_DRV80_1P2
SR111_DRV80_1P2_M#223 I/O,1.2V,SR111_DRV80_1P2
SR001_DRV80_1P2_M#224 I/O,1.2V,SR001_DRV80_1P2
SR000_DRV80_1P2_M#225 I/O,1.2V,SR000_DRV80_1P2
SR011_DRV40_1P2_M#234 I/O,1.2V,SR011_DRV40_1P2
SR010_DRV40_1P2_M#235 I/O,1.2V,SR010_DRV40_1P2
SR101_DRV40_1P2_M#236 I/O,1.2V,SR101_DRV40_1P2
SR100_DRV40_1P2_M#237 I/O,1.2V,SR100_DRV40_1P2
SR110_DRV40_1P2_M#238 I/O,1.2V,SR110_DRV40_1P2
SR111_DRV40_1P2_M#239 I/O,1.2V,SR111_DRV40_1P2
SR001_DRV40_1P2_M#240 I/O,1.2V,SR001_DRV40_1P2
SR000_DRV40_1P2_M#241 I/O,1.2V,SR000_DRV40_1P2
SR011_DRV34_1P2_M#242 I/O,1.2V,SR011_DRV34_1P2
SR010_DRV34_1P2_M#243 I/O,1.2V,SR010_DRV34_1P2
SR101_DRV34_1P2_M#244 I/O,1.2V,SR101_DRV34_1P2
SR100_DRV34_1P2_M#245 I/O,1.2V,SR100_DRV34_1P2
SR110_DRV34_1P2_M#246 I/O,1.2V,SR110_DRV34_1P2
SR111_DRV34_1P2_M#247 I/O,1.2V,SR111_DRV34_1P2
SR001_DRV34_1P2_M#248 I/O,1.2V,SR001_DRV34_1P2
SR000_DRV34_1P2_M#249 I/O,1.2V,SR000_DRV34_1P2
SR011_DRV48_1P2_M#266 I/O,1.2V,SR011_DRV48_1P2
SR010_DRV48_1P2_M#267 I/O,1.2V,SR010_DRV48_1P2
SR101_DRV48_1P2_M#268 I/O,1.2V,SR101_DRV48_1P2
SR100_DRV48_1P2_M#269 I/O,1.2V,SR100_DRV48_1P2
SR110_DRV48_1P2_M#270 I/O,1.2V,SR110_DRV48_1P2
SR111_DRV48_1P2_M#271 I/O,1.2V,SR111_DRV48_1P2
SR001_DRV48_1P2_M#272 I/O,1.2V,SR001_DRV48_1P2
SR000_DRV48_1P2_M#273 I/O,1.2V,SR000_DRV48_1P2
SR011_DRV48_1P8_M#282 I/O,1.8V,SR011_DRV48_1P8
SR010_DRV48_1P8_M#283 I/O,1.8V,SR010_DRV48_1P8
SR101_DRV48_1P8_M#284 I/O,1.8V,SR101_DRV48_1P8
SR100_DRV48_1P8_M#285 I/O,1.8V,SR100_DRV48_1P8
SR110_DRV48_1P8_M#286 I/O,1.8V,SR110_DRV48_1P8
SR111_DRV48_1P8_M#287 I/O,1.8V,SR111_DRV48_1P8
SR001_DRV48_1P8_M#288 I/O,1.8V,SR001_DRV48_1P8
SR000_DRV48_1P8_M#289 I/O,1.8V,SR000_DRV48_1P8
SR011_DRV40_1P8_M#290 I/O,1.8V,SR011_DRV40_1P8
SR010_DRV40_1P8_M#291 I/O,1.8V,SR010_DRV40_1P8
SR101_DRV40_1P8_M#292 I/O,1.8V,SR101_DRV40_1P8
SR100_DRV40_1P8_M#293 I/O,1.8V,SR100_DRV40_1P8
SR110_DRV40_1P8_M#294 I/O,1.8V,SR110_DRV40_1P8
SR111_DRV40_1P8_M#295 I/O,1.8V,SR111_DRV40_1P8
SR001_DRV40_1P8_M#296 I/O,1.8V,SR001_DRV40_1P8
SR000_DRV40_1P8_M#297 I/O,1.8V,SR000_DRV40_1P8
SR011_DRV34_1P8_M#298 I/O,1.8V,SR011_DRV34_1P8
SR010_DRV34_1P8_M#299 I/O,1.8V,SR010_DRV34_1P8
SR101_DRV34_1P8_M#300 I/O,1.8V,SR101_DRV34_1P8
SR100_DRV34_1P8_M#301 I/O,1.8V,SR100_DRV34_1P8
SR110_DRV34_1P8_M#302 I/O,1.8V,SR110_DRV34_1P8
SR111_DRV34_1P8_M#303 I/O,1.8V,SR111_DRV34_1P8
SR001_DRV34_1P8_M#304 I/O,1.8V,SR001_DRV34_1P8
SR000_DRV34_1P8_M#305 I/O,1.8V,SR000_DRV34_1P8
SR011_DRV40_1P5_M#315 I/O,1.5V,SR011_DRV40_1P5
SR010_DRV40_1P5_M#316 I/O,1.5V,SR010_DRV40_1P5
SR101_DRV40_1P5_M#317 I/O,1.5V,SR101_DRV40_1P5
SR100_DRV40_1P5_M#318 I/O,1.5V,SR100_DRV40_1P5
SR110_DRV40_1P5_M#319 I/O,1.5V,SR110_DRV40_1P5
SR111_DRV40_1P5_M#320 I/O,1.5V,SR111_DRV40_1P5
SR001_DRV40_1P5_M#321 I/O,1.5V,SR001_DRV40_1P5
SR000_DRV40_1P5_M#322 I/O,1.5V,SR000_DRV40_1P5
SR011_DRV34_1P5_M#323 I/O,1.5V,SR011_DRV34_1P5
SR010_DRV34_1P5_M#324 I/O,1.5V,SR010_DRV34_1P5
SR101_DRV34_1P5_M#325 I/O,1.5V,SR101_DRV34_1P5
SR100_DRV34_1P5_M#326 I/O,1.5V,SR100_DRV34_1P5
SR110_DRV34_1P5_M#327 I/O,1.5V,SR110_DRV34_1P5
SR111_DRV34_1P5_M#328 I/O,1.5V,SR111_DRV34_1P5
SR001_DRV34_1P5_M#329 I/O,1.5V,SR001_DRV34_1P5
SR000_DRV34_1P5_M#330 I/O,1.5V,SR000_DRV34_1P5
SR011_DRV48_1P5_M#331 I/O,1.5V,SR011_DRV48_1P5
SR010_DRV48_1P5_M#332 I/O,1.5V,SR010_DRV48_1P5
SR101_DRV48_1P5_M#333 I/O,1.5V,SR101_DRV48_1P5
SR100_DRV48_1P5_M#334 I/O,1.5V,SR100_DRV48_1P5
SR110_DRV48_1P5_M#335 I/O,1.5V,SR110_DRV48_1P5
SR111_DRV48_1P5_M#336 I/O,1.5V,SR111_DRV48_1P5
SR001_DRV48_1P5_M#337 I/O,1.5V,SR001_DRV48_1P5
SR000_DRV48_1P5_M#338 I/O,1.5V,SR000_DRV48_1P5
SR011_DRV40_1P35_M#339 I/O,1.35V,SR011_DRV40_1P35
SR010_DRV40_1P35_M#340 I/O,1.35V,SR010_DRV40_1P35
SR101_DRV40_1P35_M#341 I/O,1.35V,SR101_DRV40_1P35
SR100_DRV40_1P35_M#342 I/O,1.35V,SR100_DRV40_1P35
SR110_DRV40_1P35_M#343 I/O,1.35V,SR110_DRV40_1P35
SR111_DRV40_1P35_M#344 I/O,1.35V,SR111_DRV40_1P35
SR001_DRV40_1P35_M#345 I/O,1.35V,SR001_DRV40_1P35
SR000_DRV40_1P35_M#346 I/O,1.35V,SR000_DRV40_1P35
SR011_DRV34_1P35_M#347 I/O,1.35V,SR011_DRV34_1P35
SR010_DRV34_1P35_M#348 I/O,1.35V,SR010_DRV34_1P35
SR101_DRV34_1P35_M#349 I/O,1.35V,SR101_DRV34_1P35
SR100_DRV34_1P35_M#350 I/O,1.35V,SR100_DRV34_1P35
SR110_DRV34_1P35_M#351 I/O,1.35V,SR110_DRV34_1P35
SR111_DRV34_1P35_M#352 I/O,1.35V,SR111_DRV34_1P35
SR001_DRV34_1P35_M#353 I/O,1.35V,SR001_DRV34_1P35
SR000_DRV34_1P35_M#354 I/O,1.35V,SR000_DRV34_1P35
SR011_DRV48_1P35_M#355 I/O,1.35V,SR011_DRV48_1P35
SR010_DRV48_1P35_M#356 I/O,1.35V,SR010_DRV48_1P35
SR101_DRV48_1P35_M#357 I/O,1.35V,SR101_DRV48_1P35
SR100_DRV48_1P35_M#358 I/O,1.35V,SR100_DRV48_1P35
SR110_DRV48_1P35_M#359 I/O,1.35V,SR110_DRV48_1P35
SR111_DRV48_1P35_M#360 I/O,1.35V,SR111_DRV48_1P35
SR001_DRV48_1P35_M#361 I/O,1.35V,SR001_DRV48_1P35
SR000_DRV48_1P35_M#362 I/O,1.35V,SR000_DRV48_1P35
|   Usage OUTPUT#1.2/1.35/1.5/1.8###DDR_SEIOPB_V.PAD
|   Base model DDR_SEIOPB_V
[Model Selector] Selector_11
SR000_DRV48_1P8_M#100 I/O,1.8V,SR000_DRV48_1P8
SR011_DRV40_1P8_M#101 I/O,1.8V,SR011_DRV40_1P8
SR010_DRV40_1P8_M#102 I/O,1.8V,SR010_DRV40_1P8
SR101_DRV40_1P8_M#103 I/O,1.8V,SR101_DRV40_1P8
SR100_DRV40_1P8_M#104 I/O,1.8V,SR100_DRV40_1P8
SR110_DRV40_1P8_M#105 I/O,1.8V,SR110_DRV40_1P8
SR111_DRV40_1P8_M#106 I/O,1.8V,SR111_DRV40_1P8
SR001_DRV40_1P8_M#107 I/O,1.8V,SR001_DRV40_1P8
SR000_DRV40_1P8_M#108 I/O,1.8V,SR000_DRV40_1P8
SR011_DRV34_1P8_M#109 I/O,1.8V,SR011_DRV34_1P8
SR010_DRV34_1P8_M#110 I/O,1.8V,SR010_DRV34_1P8
SR101_DRV34_1P8_M#111 I/O,1.8V,SR101_DRV34_1P8
SR100_DRV34_1P8_M#112 I/O,1.8V,SR100_DRV34_1P8
SR110_DRV34_1P8_M#113 I/O,1.8V,SR110_DRV34_1P8
SR111_DRV34_1P8_M#114 I/O,1.8V,SR111_DRV34_1P8
SR001_DRV34_1P8_M#115 I/O,1.8V,SR001_DRV34_1P8
SR000_DRV34_1P8_M#116 I/O,1.8V,SR000_DRV34_1P8
SR011_DRV40_1P5_M#126 I/O,1.5V,SR011_DRV40_1P5
SR010_DRV40_1P5_M#127 I/O,1.5V,SR010_DRV40_1P5
SR101_DRV40_1P5_M#128 I/O,1.5V,SR101_DRV40_1P5
SR100_DRV40_1P5_M#129 I/O,1.5V,SR100_DRV40_1P5
SR011_DRV60_1P2_M#13 I/O,1.2V,SR011_DRV60_1P2
SR110_DRV40_1P5_M#130 I/O,1.5V,SR110_DRV40_1P5
SR111_DRV40_1P5_M#131 I/O,1.5V,SR111_DRV40_1P5
SR001_DRV40_1P5_M#132 I/O,1.5V,SR001_DRV40_1P5
SR000_DRV40_1P5_M#133 I/O,1.5V,SR000_DRV40_1P5
SR011_DRV34_1P5_M#134 I/O,1.5V,SR011_DRV34_1P5
SR010_DRV34_1P5_M#135 I/O,1.5V,SR010_DRV34_1P5
SR101_DRV34_1P5_M#136 I/O,1.5V,SR101_DRV34_1P5
SR100_DRV34_1P5_M#137 I/O,1.5V,SR100_DRV34_1P5
SR110_DRV34_1P5_M#138 I/O,1.5V,SR110_DRV34_1P5
SR111_DRV34_1P5_M#139 I/O,1.5V,SR111_DRV34_1P5
SR010_DRV60_1P2_M#14 I/O,1.2V,SR010_DRV60_1P2
SR001_DRV34_1P5_M#140 I/O,1.5V,SR001_DRV34_1P5
SR000_DRV34_1P5_M#141 I/O,1.5V,SR000_DRV34_1P5
SR011_DRV48_1P5_M#142 I/O,1.5V,SR011_DRV48_1P5
SR010_DRV48_1P5_M#143 I/O,1.5V,SR010_DRV48_1P5
SR101_DRV48_1P5_M#144 I/O,1.5V,SR101_DRV48_1P5
SR100_DRV48_1P5_M#145 I/O,1.5V,SR100_DRV48_1P5
SR110_DRV48_1P5_M#146 I/O,1.5V,SR110_DRV48_1P5
SR111_DRV48_1P5_M#147 I/O,1.5V,SR111_DRV48_1P5
SR001_DRV48_1P5_M#148 I/O,1.5V,SR001_DRV48_1P5
SR000_DRV48_1P5_M#149 I/O,1.5V,SR000_DRV48_1P5
SR101_DRV60_1P2_M#15 I/O,1.2V,SR101_DRV60_1P2
SR011_DRV40_1P35_M#150 I/O,1.35V,SR011_DRV40_1P35
SR010_DRV40_1P35_M#151 I/O,1.35V,SR010_DRV40_1P35
SR101_DRV40_1P35_M#152 I/O,1.35V,SR101_DRV40_1P35
SR100_DRV40_1P35_M#153 I/O,1.35V,SR100_DRV40_1P35
SR110_DRV40_1P35_M#154 I/O,1.35V,SR110_DRV40_1P35
SR111_DRV40_1P35_M#155 I/O,1.35V,SR111_DRV40_1P35
SR001_DRV40_1P35_M#156 I/O,1.35V,SR001_DRV40_1P35
SR000_DRV40_1P35_M#157 I/O,1.35V,SR000_DRV40_1P35
SR011_DRV34_1P35_M#158 I/O,1.35V,SR011_DRV34_1P35
SR010_DRV34_1P35_M#159 I/O,1.35V,SR010_DRV34_1P35
SR100_DRV60_1P2_M#16 I/O,1.2V,SR100_DRV60_1P2
SR101_DRV34_1P35_M#160 I/O,1.35V,SR101_DRV34_1P35
SR100_DRV34_1P35_M#161 I/O,1.35V,SR100_DRV34_1P35
SR110_DRV34_1P35_M#162 I/O,1.35V,SR110_DRV34_1P35
SR111_DRV34_1P35_M#163 I/O,1.35V,SR111_DRV34_1P35
SR001_DRV34_1P35_M#164 I/O,1.35V,SR001_DRV34_1P35
SR000_DRV34_1P35_M#165 I/O,1.35V,SR000_DRV34_1P35
SR011_DRV48_1P35_M#166 I/O,1.35V,SR011_DRV48_1P35
SR010_DRV48_1P35_M#167 I/O,1.35V,SR010_DRV48_1P35
SR101_DRV48_1P35_M#168 I/O,1.35V,SR101_DRV48_1P35
SR100_DRV48_1P35_M#169 I/O,1.35V,SR100_DRV48_1P35
SR110_DRV60_1P2_M#17 I/O,1.2V,SR110_DRV60_1P2
SR110_DRV48_1P35_M#170 I/O,1.35V,SR110_DRV48_1P35
SR111_DRV48_1P35_M#171 I/O,1.35V,SR111_DRV48_1P35
SR001_DRV48_1P35_M#172 I/O,1.35V,SR001_DRV48_1P35
SR000_DRV48_1P35_M#173 I/O,1.35V,SR000_DRV48_1P35
SR111_DRV60_1P2_M#18 I/O,1.2V,SR111_DRV60_1P2
SR001_DRV60_1P2_M#19 I/O,1.2V,SR001_DRV60_1P2
SR000_DRV60_1P2_M#20 I/O,1.2V,SR000_DRV60_1P2
SR011_DRV80_1P2_M#29 I/O,1.2V,SR011_DRV80_1P2
SR010_DRV80_1P2_M#30 I/O,1.2V,SR010_DRV80_1P2
SR101_DRV80_1P2_M#31 I/O,1.2V,SR101_DRV80_1P2
SR100_DRV80_1P2_M#32 I/O,1.2V,SR100_DRV80_1P2
SR110_DRV80_1P2_M#33 I/O,1.2V,SR110_DRV80_1P2
SR111_DRV80_1P2_M#34 I/O,1.2V,SR111_DRV80_1P2
SR001_DRV80_1P2_M#35 I/O,1.2V,SR001_DRV80_1P2
SR000_DRV80_1P2_M#36 I/O,1.2V,SR000_DRV80_1P2
SR011_DRV40_1P2_M#45 I/O,1.2V,SR011_DRV40_1P2
SR010_DRV40_1P2_M#46 I/O,1.2V,SR010_DRV40_1P2
SR101_DRV40_1P2_M#47 I/O,1.2V,SR101_DRV40_1P2
SR100_DRV40_1P2_M#48 I/O,1.2V,SR100_DRV40_1P2
SR110_DRV40_1P2_M#49 I/O,1.2V,SR110_DRV40_1P2
SR111_DRV40_1P2_M#50 I/O,1.2V,SR111_DRV40_1P2
SR001_DRV40_1P2_M#51 I/O,1.2V,SR001_DRV40_1P2
SR000_DRV40_1P2_M#52 I/O,1.2V,SR000_DRV40_1P2
SR011_DRV34_1P2_M#53 I/O,1.2V,SR011_DRV34_1P2
SR010_DRV34_1P2_M#54 I/O,1.2V,SR010_DRV34_1P2
SR101_DRV34_1P2_M#55 I/O,1.2V,SR101_DRV34_1P2
SR100_DRV34_1P2_M#56 I/O,1.2V,SR100_DRV34_1P2
SR110_DRV34_1P2_M#57 I/O,1.2V,SR110_DRV34_1P2
SR111_DRV34_1P2_M#58 I/O,1.2V,SR111_DRV34_1P2
SR001_DRV34_1P2_M#59 I/O,1.2V,SR001_DRV34_1P2
SR000_DRV34_1P2_M#60 I/O,1.2V,SR000_DRV34_1P2
SR011_DRV48_1P2_M#77 I/O,1.2V,SR011_DRV48_1P2
SR010_DRV48_1P2_M#78 I/O,1.2V,SR010_DRV48_1P2
SR101_DRV48_1P2_M#79 I/O,1.2V,SR101_DRV48_1P2
SR100_DRV48_1P2_M#80 I/O,1.2V,SR100_DRV48_1P2
SR110_DRV48_1P2_M#81 I/O,1.2V,SR110_DRV48_1P2
SR111_DRV48_1P2_M#82 I/O,1.2V,SR111_DRV48_1P2
SR001_DRV48_1P2_M#83 I/O,1.2V,SR001_DRV48_1P2
SR000_DRV48_1P2_M#84 I/O,1.2V,SR000_DRV48_1P2
SR011_DRV48_1P8_M#93 I/O,1.8V,SR011_DRV48_1P8
SR010_DRV48_1P8_M#94 I/O,1.8V,SR010_DRV48_1P8
SR101_DRV48_1P8_M#95 I/O,1.8V,SR101_DRV48_1P8
SR100_DRV48_1P8_M#96 I/O,1.8V,SR100_DRV48_1P8
SR110_DRV48_1P8_M#97 I/O,1.8V,SR110_DRV48_1P8
SR111_DRV48_1P8_M#98 I/O,1.8V,SR111_DRV48_1P8
SR001_DRV48_1P8_M#99 I/O,1.8V,SR001_DRV48_1P8
|   Usage OUTPUT#1.2/1.35/1.5/1.8###DDR_DIFFIOPB_V.PADN
|   Base model DDR_DIFFIOPB_V
[Model Selector] Selector_12
SR011_DRV60_1P2_M#202 I/O,1.2V,SR011_DRV60_1P2
SR010_DRV60_1P2_M#203 I/O,1.2V,SR010_DRV60_1P2
SR101_DRV60_1P2_M#204 I/O,1.2V,SR101_DRV60_1P2
SR100_DRV60_1P2_M#205 I/O,1.2V,SR100_DRV60_1P2
SR110_DRV60_1P2_M#206 I/O,1.2V,SR110_DRV60_1P2
SR111_DRV60_1P2_M#207 I/O,1.2V,SR111_DRV60_1P2
SR001_DRV60_1P2_M#208 I/O,1.2V,SR001_DRV60_1P2
SR000_DRV60_1P2_M#209 I/O,1.2V,SR000_DRV60_1P2
SR011_DRV80_1P2_M#218 I/O,1.2V,SR011_DRV80_1P2
SR010_DRV80_1P2_M#219 I/O,1.2V,SR010_DRV80_1P2
SR101_DRV80_1P2_M#220 I/O,1.2V,SR101_DRV80_1P2
SR100_DRV80_1P2_M#221 I/O,1.2V,SR100_DRV80_1P2
SR110_DRV80_1P2_M#222 I/O,1.2V,SR110_DRV80_1P2
SR111_DRV80_1P2_M#223 I/O,1.2V,SR111_DRV80_1P2
SR001_DRV80_1P2_M#224 I/O,1.2V,SR001_DRV80_1P2
SR000_DRV80_1P2_M#225 I/O,1.2V,SR000_DRV80_1P2
SR011_DRV40_1P2_M#234 I/O,1.2V,SR011_DRV40_1P2
SR010_DRV40_1P2_M#235 I/O,1.2V,SR010_DRV40_1P2
SR101_DRV40_1P2_M#236 I/O,1.2V,SR101_DRV40_1P2
SR100_DRV40_1P2_M#237 I/O,1.2V,SR100_DRV40_1P2
SR110_DRV40_1P2_M#238 I/O,1.2V,SR110_DRV40_1P2
SR111_DRV40_1P2_M#239 I/O,1.2V,SR111_DRV40_1P2
SR001_DRV40_1P2_M#240 I/O,1.2V,SR001_DRV40_1P2
SR000_DRV40_1P2_M#241 I/O,1.2V,SR000_DRV40_1P2
SR011_DRV34_1P2_M#242 I/O,1.2V,SR011_DRV34_1P2
SR010_DRV34_1P2_M#243 I/O,1.2V,SR010_DRV34_1P2
SR101_DRV34_1P2_M#244 I/O,1.2V,SR101_DRV34_1P2
SR100_DRV34_1P2_M#245 I/O,1.2V,SR100_DRV34_1P2
SR110_DRV34_1P2_M#246 I/O,1.2V,SR110_DRV34_1P2
SR111_DRV34_1P2_M#247 I/O,1.2V,SR111_DRV34_1P2
SR001_DRV34_1P2_M#248 I/O,1.2V,SR001_DRV34_1P2
SR000_DRV34_1P2_M#249 I/O,1.2V,SR000_DRV34_1P2
SR011_DRV48_1P2_M#266 I/O,1.2V,SR011_DRV48_1P2
SR010_DRV48_1P2_M#267 I/O,1.2V,SR010_DRV48_1P2
SR101_DRV48_1P2_M#268 I/O,1.2V,SR101_DRV48_1P2
SR100_DRV48_1P2_M#269 I/O,1.2V,SR100_DRV48_1P2
SR110_DRV48_1P2_M#270 I/O,1.2V,SR110_DRV48_1P2
SR111_DRV48_1P2_M#271 I/O,1.2V,SR111_DRV48_1P2
SR001_DRV48_1P2_M#272 I/O,1.2V,SR001_DRV48_1P2
SR000_DRV48_1P2_M#273 I/O,1.2V,SR000_DRV48_1P2
SR011_DRV48_1P8_M#282 I/O,1.8V,SR011_DRV48_1P8
SR010_DRV48_1P8_M#283 I/O,1.8V,SR010_DRV48_1P8
SR101_DRV48_1P8_M#284 I/O,1.8V,SR101_DRV48_1P8
SR100_DRV48_1P8_M#285 I/O,1.8V,SR100_DRV48_1P8
SR110_DRV48_1P8_M#286 I/O,1.8V,SR110_DRV48_1P8
SR111_DRV48_1P8_M#287 I/O,1.8V,SR111_DRV48_1P8
SR001_DRV48_1P8_M#288 I/O,1.8V,SR001_DRV48_1P8
SR000_DRV48_1P8_M#289 I/O,1.8V,SR000_DRV48_1P8
SR011_DRV40_1P8_M#290 I/O,1.8V,SR011_DRV40_1P8
SR010_DRV40_1P8_M#291 I/O,1.8V,SR010_DRV40_1P8
SR101_DRV40_1P8_M#292 I/O,1.8V,SR101_DRV40_1P8
SR100_DRV40_1P8_M#293 I/O,1.8V,SR100_DRV40_1P8
SR110_DRV40_1P8_M#294 I/O,1.8V,SR110_DRV40_1P8
SR111_DRV40_1P8_M#295 I/O,1.8V,SR111_DRV40_1P8
SR001_DRV40_1P8_M#296 I/O,1.8V,SR001_DRV40_1P8
SR000_DRV40_1P8_M#297 I/O,1.8V,SR000_DRV40_1P8
SR011_DRV34_1P8_M#298 I/O,1.8V,SR011_DRV34_1P8
SR010_DRV34_1P8_M#299 I/O,1.8V,SR010_DRV34_1P8
SR101_DRV34_1P8_M#300 I/O,1.8V,SR101_DRV34_1P8
SR100_DRV34_1P8_M#301 I/O,1.8V,SR100_DRV34_1P8
SR110_DRV34_1P8_M#302 I/O,1.8V,SR110_DRV34_1P8
SR111_DRV34_1P8_M#303 I/O,1.8V,SR111_DRV34_1P8
SR001_DRV34_1P8_M#304 I/O,1.8V,SR001_DRV34_1P8
SR000_DRV34_1P8_M#305 I/O,1.8V,SR000_DRV34_1P8
SR011_DRV40_1P5_M#315 I/O,1.5V,SR011_DRV40_1P5
SR010_DRV40_1P5_M#316 I/O,1.5V,SR010_DRV40_1P5
SR101_DRV40_1P5_M#317 I/O,1.5V,SR101_DRV40_1P5
SR100_DRV40_1P5_M#318 I/O,1.5V,SR100_DRV40_1P5
SR110_DRV40_1P5_M#319 I/O,1.5V,SR110_DRV40_1P5
SR111_DRV40_1P5_M#320 I/O,1.5V,SR111_DRV40_1P5
SR001_DRV40_1P5_M#321 I/O,1.5V,SR001_DRV40_1P5
SR000_DRV40_1P5_M#322 I/O,1.5V,SR000_DRV40_1P5
SR011_DRV34_1P5_M#323 I/O,1.5V,SR011_DRV34_1P5
SR010_DRV34_1P5_M#324 I/O,1.5V,SR010_DRV34_1P5
SR101_DRV34_1P5_M#325 I/O,1.5V,SR101_DRV34_1P5
SR100_DRV34_1P5_M#326 I/O,1.5V,SR100_DRV34_1P5
SR110_DRV34_1P5_M#327 I/O,1.5V,SR110_DRV34_1P5
SR111_DRV34_1P5_M#328 I/O,1.5V,SR111_DRV34_1P5
SR001_DRV34_1P5_M#329 I/O,1.5V,SR001_DRV34_1P5
SR000_DRV34_1P5_M#330 I/O,1.5V,SR000_DRV34_1P5
SR011_DRV48_1P5_M#331 I/O,1.5V,SR011_DRV48_1P5
SR010_DRV48_1P5_M#332 I/O,1.5V,SR010_DRV48_1P5
SR101_DRV48_1P5_M#333 I/O,1.5V,SR101_DRV48_1P5
SR100_DRV48_1P5_M#334 I/O,1.5V,SR100_DRV48_1P5
SR110_DRV48_1P5_M#335 I/O,1.5V,SR110_DRV48_1P5
SR111_DRV48_1P5_M#336 I/O,1.5V,SR111_DRV48_1P5
SR001_DRV48_1P5_M#337 I/O,1.5V,SR001_DRV48_1P5
SR000_DRV48_1P5_M#338 I/O,1.5V,SR000_DRV48_1P5
SR011_DRV40_1P35_M#339 I/O,1.35V,SR011_DRV40_1P35
SR010_DRV40_1P35_M#340 I/O,1.35V,SR010_DRV40_1P35
SR101_DRV40_1P35_M#341 I/O,1.35V,SR101_DRV40_1P35
SR100_DRV40_1P35_M#342 I/O,1.35V,SR100_DRV40_1P35
SR110_DRV40_1P35_M#343 I/O,1.35V,SR110_DRV40_1P35
SR111_DRV40_1P35_M#344 I/O,1.35V,SR111_DRV40_1P35
SR001_DRV40_1P35_M#345 I/O,1.35V,SR001_DRV40_1P35
SR000_DRV40_1P35_M#346 I/O,1.35V,SR000_DRV40_1P35
SR011_DRV34_1P35_M#347 I/O,1.35V,SR011_DRV34_1P35
SR010_DRV34_1P35_M#348 I/O,1.35V,SR010_DRV34_1P35
SR101_DRV34_1P35_M#349 I/O,1.35V,SR101_DRV34_1P35
SR100_DRV34_1P35_M#350 I/O,1.35V,SR100_DRV34_1P35
SR110_DRV34_1P35_M#351 I/O,1.35V,SR110_DRV34_1P35
SR111_DRV34_1P35_M#352 I/O,1.35V,SR111_DRV34_1P35
SR001_DRV34_1P35_M#353 I/O,1.35V,SR001_DRV34_1P35
SR000_DRV34_1P35_M#354 I/O,1.35V,SR000_DRV34_1P35
SR011_DRV48_1P35_M#355 I/O,1.35V,SR011_DRV48_1P35
SR010_DRV48_1P35_M#356 I/O,1.35V,SR010_DRV48_1P35
SR101_DRV48_1P35_M#357 I/O,1.35V,SR101_DRV48_1P35
SR100_DRV48_1P35_M#358 I/O,1.35V,SR100_DRV48_1P35
SR110_DRV48_1P35_M#359 I/O,1.35V,SR110_DRV48_1P35
SR111_DRV48_1P35_M#360 I/O,1.35V,SR111_DRV48_1P35
SR001_DRV48_1P35_M#361 I/O,1.35V,SR001_DRV48_1P35
SR000_DRV48_1P35_M#362 I/O,1.35V,SR000_DRV48_1P35
|   Usage I/O#1.2/1.35/1.5/1.8###DDR_DIFFIOPB_V.PADN
|   Base model DDR_DIFFIOPB_V
[Model Selector] Selector_13
SR011_DRV60_1P2_M#202 I/O,1.2V,SR011_DRV60_1P2
SR010_DRV60_1P2_M#203 I/O,1.2V,SR010_DRV60_1P2
SR101_DRV60_1P2_M#204 I/O,1.2V,SR101_DRV60_1P2
SR100_DRV60_1P2_M#205 I/O,1.2V,SR100_DRV60_1P2
SR110_DRV60_1P2_M#206 I/O,1.2V,SR110_DRV60_1P2
SR111_DRV60_1P2_M#207 I/O,1.2V,SR111_DRV60_1P2
SR001_DRV60_1P2_M#208 I/O,1.2V,SR001_DRV60_1P2
SR000_DRV60_1P2_M#209 I/O,1.2V,SR000_DRV60_1P2
SR011_DRV80_1P2_M#218 I/O,1.2V,SR011_DRV80_1P2
SR010_DRV80_1P2_M#219 I/O,1.2V,SR010_DRV80_1P2
SR101_DRV80_1P2_M#220 I/O,1.2V,SR101_DRV80_1P2
SR100_DRV80_1P2_M#221 I/O,1.2V,SR100_DRV80_1P2
SR110_DRV80_1P2_M#222 I/O,1.2V,SR110_DRV80_1P2
SR111_DRV80_1P2_M#223 I/O,1.2V,SR111_DRV80_1P2
SR001_DRV80_1P2_M#224 I/O,1.2V,SR001_DRV80_1P2
SR000_DRV80_1P2_M#225 I/O,1.2V,SR000_DRV80_1P2
SR011_DRV40_1P2_M#234 I/O,1.2V,SR011_DRV40_1P2
SR010_DRV40_1P2_M#235 I/O,1.2V,SR010_DRV40_1P2
SR101_DRV40_1P2_M#236 I/O,1.2V,SR101_DRV40_1P2
SR100_DRV40_1P2_M#237 I/O,1.2V,SR100_DRV40_1P2
SR110_DRV40_1P2_M#238 I/O,1.2V,SR110_DRV40_1P2
SR111_DRV40_1P2_M#239 I/O,1.2V,SR111_DRV40_1P2
SR001_DRV40_1P2_M#240 I/O,1.2V,SR001_DRV40_1P2
SR000_DRV40_1P2_M#241 I/O,1.2V,SR000_DRV40_1P2
SR011_DRV34_1P2_M#242 I/O,1.2V,SR011_DRV34_1P2
SR010_DRV34_1P2_M#243 I/O,1.2V,SR010_DRV34_1P2
SR101_DRV34_1P2_M#244 I/O,1.2V,SR101_DRV34_1P2
SR100_DRV34_1P2_M#245 I/O,1.2V,SR100_DRV34_1P2
SR110_DRV34_1P2_M#246 I/O,1.2V,SR110_DRV34_1P2
SR111_DRV34_1P2_M#247 I/O,1.2V,SR111_DRV34_1P2
SR001_DRV34_1P2_M#248 I/O,1.2V,SR001_DRV34_1P2
SR000_DRV34_1P2_M#249 I/O,1.2V,SR000_DRV34_1P2
SR011_DRV48_1P2_M#266 I/O,1.2V,SR011_DRV48_1P2
SR010_DRV48_1P2_M#267 I/O,1.2V,SR010_DRV48_1P2
SR101_DRV48_1P2_M#268 I/O,1.2V,SR101_DRV48_1P2
SR100_DRV48_1P2_M#269 I/O,1.2V,SR100_DRV48_1P2
SR110_DRV48_1P2_M#270 I/O,1.2V,SR110_DRV48_1P2
SR111_DRV48_1P2_M#271 I/O,1.2V,SR111_DRV48_1P2
SR001_DRV48_1P2_M#272 I/O,1.2V,SR001_DRV48_1P2
SR000_DRV48_1P2_M#273 I/O,1.2V,SR000_DRV48_1P2
SR011_DRV48_1P8_M#282 I/O,1.8V,SR011_DRV48_1P8
SR010_DRV48_1P8_M#283 I/O,1.8V,SR010_DRV48_1P8
SR101_DRV48_1P8_M#284 I/O,1.8V,SR101_DRV48_1P8
SR100_DRV48_1P8_M#285 I/O,1.8V,SR100_DRV48_1P8
SR110_DRV48_1P8_M#286 I/O,1.8V,SR110_DRV48_1P8
SR111_DRV48_1P8_M#287 I/O,1.8V,SR111_DRV48_1P8
SR001_DRV48_1P8_M#288 I/O,1.8V,SR001_DRV48_1P8
SR000_DRV48_1P8_M#289 I/O,1.8V,SR000_DRV48_1P8
SR011_DRV40_1P8_M#290 I/O,1.8V,SR011_DRV40_1P8
SR010_DRV40_1P8_M#291 I/O,1.8V,SR010_DRV40_1P8
SR101_DRV40_1P8_M#292 I/O,1.8V,SR101_DRV40_1P8
SR100_DRV40_1P8_M#293 I/O,1.8V,SR100_DRV40_1P8
SR110_DRV40_1P8_M#294 I/O,1.8V,SR110_DRV40_1P8
SR111_DRV40_1P8_M#295 I/O,1.8V,SR111_DRV40_1P8
SR001_DRV40_1P8_M#296 I/O,1.8V,SR001_DRV40_1P8
SR000_DRV40_1P8_M#297 I/O,1.8V,SR000_DRV40_1P8
SR011_DRV34_1P8_M#298 I/O,1.8V,SR011_DRV34_1P8
SR010_DRV34_1P8_M#299 I/O,1.8V,SR010_DRV34_1P8
SR101_DRV34_1P8_M#300 I/O,1.8V,SR101_DRV34_1P8
SR100_DRV34_1P8_M#301 I/O,1.8V,SR100_DRV34_1P8
SR110_DRV34_1P8_M#302 I/O,1.8V,SR110_DRV34_1P8
SR111_DRV34_1P8_M#303 I/O,1.8V,SR111_DRV34_1P8
SR001_DRV34_1P8_M#304 I/O,1.8V,SR001_DRV34_1P8
SR000_DRV34_1P8_M#305 I/O,1.8V,SR000_DRV34_1P8
DDR3_ODT_80_1P5_M#306 INPUT,1.5V,DDR3_ODT_80_1P5
DDR3_ODT_60_1P5_M#307 INPUT,1.5V,DDR3_ODT_60_1P5
DDR3_ODT_120_1P5_M#308 INPUT,1.5V,DDR3_ODT_120_1P5
DDR3L_ODT_80_1P35_M#309 INPUT,1.35V,DDR3L_ODT_80_1P35
DDR3L_ODT_60_1P35_M#310 INPUT,1.35V,DDR3L_ODT_60_1P35
DDR3L_ODT_120_1P35_M#311 INPUT,1.35V,DDR3L_ODT_120_1P35
DDR2_ODT_120_1P8_M#312 INPUT,1.8V,DDR2_ODT_120_1P8
DDR2_ODT_80_1P8_M#313 INPUT,1.8V,DDR2_ODT_80_1P8
DDR2_ODT_60_1P8_M#314 INPUT,1.8V,DDR2_ODT_60_1P8
SR011_DRV40_1P5_M#315 I/O,1.5V,SR011_DRV40_1P5
SR010_DRV40_1P5_M#316 I/O,1.5V,SR010_DRV40_1P5
SR101_DRV40_1P5_M#317 I/O,1.5V,SR101_DRV40_1P5
SR100_DRV40_1P5_M#318 I/O,1.5V,SR100_DRV40_1P5
SR110_DRV40_1P5_M#319 I/O,1.5V,SR110_DRV40_1P5
SR111_DRV40_1P5_M#320 I/O,1.5V,SR111_DRV40_1P5
SR001_DRV40_1P5_M#321 I/O,1.5V,SR001_DRV40_1P5
SR000_DRV40_1P5_M#322 I/O,1.5V,SR000_DRV40_1P5
SR011_DRV34_1P5_M#323 I/O,1.5V,SR011_DRV34_1P5
SR010_DRV34_1P5_M#324 I/O,1.5V,SR010_DRV34_1P5
SR101_DRV34_1P5_M#325 I/O,1.5V,SR101_DRV34_1P5
SR100_DRV34_1P5_M#326 I/O,1.5V,SR100_DRV34_1P5
SR110_DRV34_1P5_M#327 I/O,1.5V,SR110_DRV34_1P5
SR111_DRV34_1P5_M#328 I/O,1.5V,SR111_DRV34_1P5
SR001_DRV34_1P5_M#329 I/O,1.5V,SR001_DRV34_1P5
SR000_DRV34_1P5_M#330 I/O,1.5V,SR000_DRV34_1P5
SR011_DRV48_1P5_M#331 I/O,1.5V,SR011_DRV48_1P5
SR010_DRV48_1P5_M#332 I/O,1.5V,SR010_DRV48_1P5
SR101_DRV48_1P5_M#333 I/O,1.5V,SR101_DRV48_1P5
SR100_DRV48_1P5_M#334 I/O,1.5V,SR100_DRV48_1P5
SR110_DRV48_1P5_M#335 I/O,1.5V,SR110_DRV48_1P5
SR111_DRV48_1P5_M#336 I/O,1.5V,SR111_DRV48_1P5
SR001_DRV48_1P5_M#337 I/O,1.5V,SR001_DRV48_1P5
SR000_DRV48_1P5_M#338 I/O,1.5V,SR000_DRV48_1P5
SR011_DRV40_1P35_M#339 I/O,1.35V,SR011_DRV40_1P35
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| Models and submodels in the file (282): IQ1833_V_10P_1P8_M#1 (Input), IQ1833_V_5P_1P8_M#2 (Input), IQ1833_V_10P_3P3_M#3 (Input), IQ1833_V_5P_3P3_M#4 (Input), CAMERARX_ADDON_HSRX_M#7 (Input), CAMERARX_ADDON_LPRX_M#8 (Input), CAMERARX_ADDON_ULPRX_M#9 (Input), CAMERARX_ADDON_PD_ON_M#10 (Input), CAMERARX_ADDON_PU_ON_M#11 (Input), CAMERARX_ADDON_PUPD0_M#12 (Input), SR011_DRV60_1P2_M#13 (I/O), SR010_DRV60_1P2_M#14 (I/O), SR101_DRV60_1P2_M#15 (I/O), SR100_DRV60_1P2_M#16 (I/O), SR110_DRV60_1P2_M#17 (I/O), SR111_DRV60_1P2_M#18 (I/O), SR001_DRV60_1P2_M#19 (I/O), SR000_DRV60_1P2_M#20 (I/O), SR011_DRV80_1P2_M#29 (I/O), SR010_DRV80_1P2_M#30 (I/O), SR101_DRV80_1P2_M#31 (I/O), SR100_DRV80_1P2_M#32 (I/O), SR110_DRV80_1P2_M#33 (I/O), SR111_DRV80_1P2_M#34 (I/O), SR001_DRV80_1P2_M#35 (I/O), SR000_DRV80_1P2_M#36 (I/O), SR011_DRV40_1P2_M#45 (I/O), SR010_DRV40_1P2_M#46 (I/O), SR101_DRV40_1P2_M#47 (I/O), SR100_DRV40_1P2_M#48 (I/O), SR110_DRV40_1P2_M#49 (I/O), SR111_DRV40_1P2_M#50 (I/O), SR001_DRV40_1P2_M#51 (I/O), SR000_DRV40_1P2_M#52 (I/O), SR011_DRV34_1P2_M#53 (I/O), SR010_DRV34_1P2_M#54 (I/O), SR101_DRV34_1P2_M#55 (I/O), SR100_DRV34_1P2_M#56 (I/O), SR110_DRV34_1P2_M#57 (I/O), SR111_DRV34_1P2_M#58 (I/O), SR001_DRV34_1P2_M#59 (I/O), SR000_DRV34_1P2_M#60 (I/O), SR011_DRV48_1P2_M#77 (I/O), SR010_DRV48_1P2_M#78 (I/O), SR101_DRV48_1P2_M#79 (I/O), SR100_DRV48_1P2_M#80 (I/O), SR110_DRV48_1P2_M#81 (I/O), SR111_DRV48_1P2_M#82 (I/O), SR001_DRV48_1P2_M#83 (I/O), SR000_DRV48_1P2_M#84 (I/O), SR011_DRV48_1P8_M#93 (I/O), SR010_DRV48_1P8_M#94 (I/O), SR101_DRV48_1P8_M#95 (I/O), SR100_DRV48_1P8_M#96 (I/O), SR110_DRV48_1P8_M#97 (I/O), SR111_DRV48_1P8_M#98 (I/O), SR001_DRV48_1P8_M#99 (I/O), SR000_DRV48_1P8_M#100 (I/O), SR011_DRV40_1P8_M#101 (I/O), SR010_DRV40_1P8_M#102 (I/O), SR101_DRV40_1P8_M#103 (I/O), SR100_DRV40_1P8_M#104 (I/O), SR110_DRV40_1P8_M#105 (I/O), SR111_DRV40_1P8_M#106 (I/O), SR001_DRV40_1P8_M#107 (I/O), SR000_DRV40_1P8_M#108 (I/O), SR011_DRV34_1P8_M#109 (I/O), SR010_DRV34_1P8_M#110 (I/O), SR101_DRV34_1P8_M#111 (I/O), SR100_DRV34_1P8_M#112 (I/O), SR110_DRV34_1P8_M#113 (I/O), SR111_DRV34_1P8_M#114 (I/O), SR001_DRV34_1P8_M#115 (I/O), SR000_DRV34_1P8_M#116 (I/O), DDR3_ODT_80_1P5_M#117 (Input), DDR3_ODT_60_1P5_M#118 (Input), DDR3_ODT_120_1P5_M#119 (Input), DDR3L_ODT_80_1P35_M#120 (Input), DDR3L_ODT_60_1P35_M#121 (Input), DDR3L_ODT_120_1P35_M#122 (Input)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
